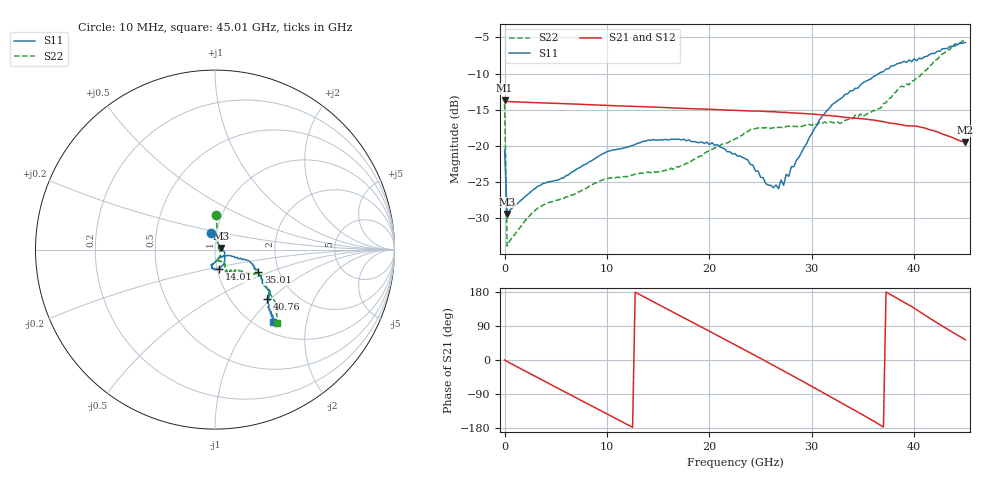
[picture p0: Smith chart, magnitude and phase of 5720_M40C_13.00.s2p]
! Device:  ADRF5720
! Description: 0.5dB LSB GaAs MMIC 6-bit Digital Attenuator
! Frequency:  0.000009 -  40 GHz
! Ports:
!	RF1	= Port 1
!	RF2	= Port 2
! Vdd:  3.3 Volt
! Vss:  -3.3 Volt
! Control:  0/3.3 Volt
! State:  13.00 dB attenuation
! Data:  The device was measured using G-S-G Probes on a matrix board.
!  Data was collected using an calibrated 4 port network analyzer.
!  The reference plane for this measurement is at the launchers.
! Note:  Analog Devices supplies this data as a sample of measured data
!  for this product.  Your particular data for this product may vary.
!  Data was taken at -40 degrees C.
!  Analog Devices reserves the right to change this data at anytime.
# GHZ S DB R 45.0
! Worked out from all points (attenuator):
!   181 points, 10 MHz to 45.01 GHz, reference 45 ohm
!   highest |S21| = -13.70 dB at 10 MHz (marker M1); lowest = -19.5 dB at 45.01 GHz (marker M2)
!   lowest |S11| = -29.4 dB at 260 MHz (marker M3), VSWR 1.07, Z = 48 + j0.828 ohm
!   |S11| at or under -10 dB: start of sweep to 36.58 GHz
!   |S22| runs from -33.8 to -5.4 dB; largest |S21 - S12| = 0.00075
!   S11 on the Smith chart (normalised r, x): 10 MHz: 0.95, +0.18; 14.01 GHz: 1.02, -0.22; 35.01 GHz: 1.57, -0.43; 40.76 GHz: 1.45, -0.95; 45.01 GHz: 1.19, -1.30
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0.01  -20.55 102.0  -13.70 0.2  -13.72 0.2  -14.23 88.3
0.26  -29.40 14.7  -13.87 -3.9  -13.89 -3.9  -33.84 22.2
3.26  -25.56 -12.4  -14.03 -46.9  -14.06 -47.0  -28.56 -30.4
7.76  -22.60 -42.9  -14.27 -110.6  -14.29 -110.6  -25.97 -64.2
11.01  -20.46 -59.7  -14.46 -156.4  -14.47 -156.5  -24.31 -73.1
14.01  -19.18 -77.8  -14.61 161.2  -14.63 161.1  -23.60 -74.9
15.26  -19.14 -82.9  -14.67 143.4  -14.69 143.3  -23.54 -71.7
19.01  -19.55 -97.1  -14.88 90.1  -14.90 90.0  -21.44 -59.2
22.76  -21.40 -103.6  -15.10 36.5  -15.12 36.5  -18.89 -60.2
24.01  -22.56 -93.7  -15.18 18.7  -15.20 18.6  -17.72 -61.3
26.76  -25.91 -50.8  -15.34 -21.5  -15.36 -21.7  -17.40 -62.4
27.01  -24.70 -46.2  -15.35 -25.0  -15.37 -25.2  -17.45 -64.2
27.26  -25.44 -43.0  -15.35 -28.7  -15.37 -28.9  -17.47 -62.8
27.51  -23.91 -37.1  -15.36 -32.5  -15.38 -32.6  -17.31 -64.0
27.76  -24.19 -33.5  -15.41 -36.2  -15.43 -36.4  -17.29 -62.5
30.26  -17.64 -19.1  -15.62 -73.4  -15.64 -73.5  -16.90 -62.3
32.01  -14.28 -18.8  -15.85 -99.6  -15.87 -99.8  -16.75 -56.2
35.01  -11.28 -27.5  -16.27 -145.0  -16.29 -145.1  -15.93 -45.0
37.76  -8.96 -36.9  -16.86 171.8  -16.88 171.6  -13.32 -37.0
40.76  -7.97 -43.5  -17.44 123.8  -17.48 123.6  -10.02 -31.8
43.76  -6.28 -48.7  -18.84 73.1  -18.87 73.0  -6.06 -44.7
45.01  -5.72 -51.0  -19.49 53.5  -19.53 53.3  -5.43 -50.0
